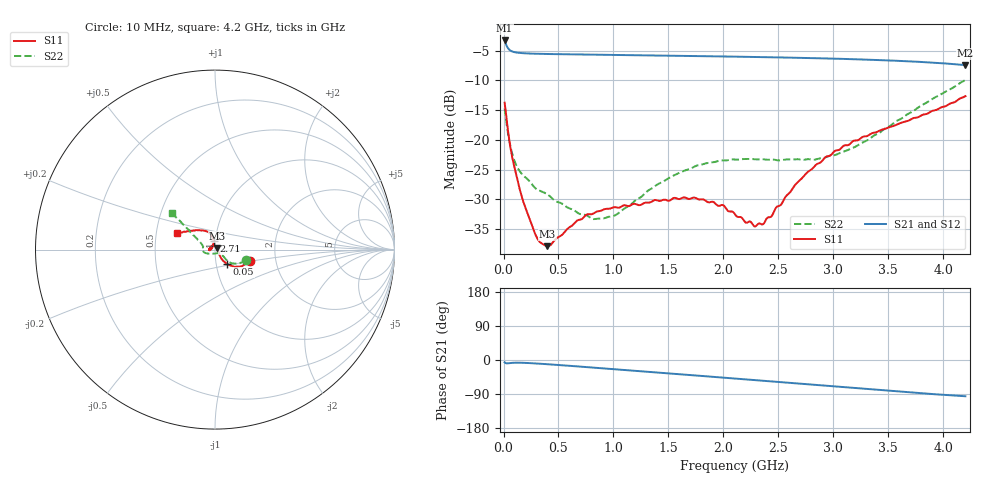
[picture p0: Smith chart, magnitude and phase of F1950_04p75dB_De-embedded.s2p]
! Integrated Device Technology
! Corporate Headquarters
! 6024 Silver Creek Valley Road
! San Jose, CA 95138  USA
! Phone:  1-408-284-8200
! Toll Free:  1-800-223-1366
! Webpage:  http://www.idt.com/
! Timing and RF Division
! 515 Groton Road, Suite 102
! Westford, MA 01886-6024
! Device:  F1950
! Description: 7-bit 0.25 dB Digital Step Attenuator
! Frequency:  150.0 -  4000.00 MHz
! Package:  4x4 mm Thin QFN Plastic Package: 24 pin
! Ports:  2 RF, 12 DC
!  Pin  1  = D0
!  Pin  2  = VDD
!  Pin  3  = Vmode
!  Pin  4  = GND
!  Pin  5  = RF1  =  Port 1
!  Pin  6  = GND
!  Pin  7  = GND
!  Pin  8  = GND
!  Pin  9  = GND
!  Pin 10  = GND
!  Pin 11  = GND
!  Pin 12  = GND
!  Pin 13  = GND
!  Pin 14  = RF2  =  Port 2
!  Pin 15  = GND
!  Pin 16  = LE
!  Pin 17  = CLK
!  Pin 18  = DATE
!  Pin 19  = D6
!  Pin 20  = D5
!  Pin 21  = D4
!  Pin 22  = D3
!  Pin 23  = D2
!  Pin 24  = D1
! State:  19
! Atten State:  4.75 dB
! Voltage:  +5.00 Volts
! Current:  Not Measured mA
! Data:  The device was measured on a the F195X evaluation board which has
!  individual transmission lines to the RF pins.  Data was collected
!  using a calibrated network analyzer.  The evaluation board was
!  de-embedded using a TRL calibration technique.
!  The reference plane is the edge of the package pin.
! Misc:  Board 2019
!  Action Tracker AT0250
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# GHz S dB R 50
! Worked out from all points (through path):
!   420 points, 10 MHz to 4.2 GHz, reference 50 ohm
!   highest |S21| = -3.30 dB at 10 MHz (marker M1); lowest = -7.4 dB at 4.2 GHz (marker M2)
!   group delay of S21, straight-line fit = 62.1 ps
!   lowest |S11| = -37.9 dB at 400 MHz (marker M3), VSWR 1.03, Z = 51.1 + j0.703 ohm
!   |S11| at or under -10 dB: start of sweep to end of sweep
!   |S22| runs from -33.3 to -10.0 dB; largest |S21 - S12| = 0.0018
!   S11 on the Smith chart (normalised r, x): 10 MHz: 1.47, -0.20; 50 MHz: 1.13, -0.18; 2.71 GHz: 0.98, +0.09; 4.2 GHz: 0.64, +0.13
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0.01  -13.76 -18.8  -3.30 -6.0  -3.30 -6.0  -14.74 -19.2
0.05  -19.76 -50.2  -4.81 -8.4  -4.81 -8.5  -19.93 -41.7
0.08  -23.02 -54.3  -5.16 -7.5  -5.16 -7.5  -22.39 -41.2
0.11  -25.40 -53.9  -5.31 -7.1  -5.30 -7.1  -24.03 -38.8
0.2  -31.45 -38.1  -5.47 -7.6  -5.46 -7.7  -26.32 -38.7
0.31  -36.67 -4.7  -5.54 -9.4  -5.54 -9.4  -28.41 -39.1
0.4  -37.88 32.6  -5.58 -11.1  -5.57 -11.2  -29.18 -39.5
0.71  -33.36 100.6  -5.66 -17.7  -5.65 -17.8  -32.54 -59.1
0.83  -32.25 111.5  -5.68 -20.3  -5.68 -20.4  -33.33 -75.1
1.01  -31.33 129.1  -5.73 -24.3  -5.73 -24.4  -32.75 -103.4
1.41  -30.26 167.8  -5.82 -33.2  -5.82 -33.4  -27.40 -147.4
1.74  -29.73 -174.3  -5.91 -40.7  -5.91 -40.8  -24.47 -163.5
1.99  -30.96 -174.8  -5.98 -46.4  -5.98 -46.5  -23.47 -171.6
2.11  -32.65 -179.1  -6.02 -49.1  -6.02 -49.2  -23.34 -175.8
2.28  -34.56 154.6  -6.08 -52.9  -6.08 -53.1  -23.28 179.6
2.36  -34.19 136.8  -6.11 -54.8  -6.11 -54.9  -23.27 177.4
2.71  -26.54 99.9  -6.23 -62.8  -6.22 -62.9  -23.36 168.8
2.81  -24.82 98.3  -6.27 -65.0  -6.27 -65.2  -23.37 165.8
3.01  -21.91 102.2  -6.36 -69.7  -6.36 -69.9  -22.58 160.9
3.18  -20.20 107.2  -6.45 -73.7  -6.45 -73.9  -21.33 155.4
3.51  -17.86 123.3  -6.66 -81.2  -6.66 -81.4  -17.73 147.6
4.2  -12.67 156.3  -7.45 -95.7  -7.44 -95.9  -9.96 139.4
